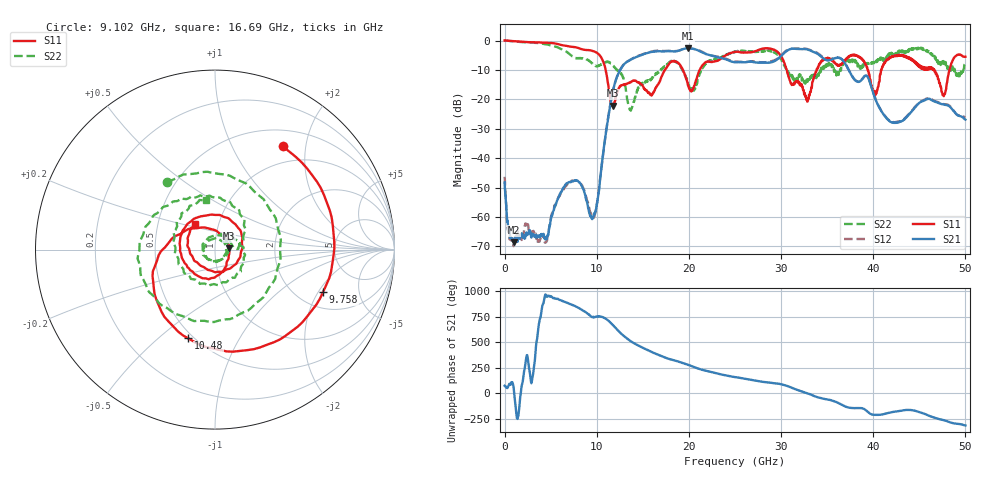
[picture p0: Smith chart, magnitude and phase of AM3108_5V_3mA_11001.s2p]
# Hz S DB R 50.0
!freq dBS11 angS11 dBS21 angS21 dBS12 angS12 dBS22 angS22
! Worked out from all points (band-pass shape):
!   1601 points, 10 MHz to 50 GHz, reference 50 ohm
!   highest |S21| = -2.67 dB at 19.91 GHz (marker M1); lowest = -68.6 dB at 978.6 MHz (marker M2)
!   |S21| within 3 dB of the highest: 14.24 GHz to 23.08 GHz (8.833 GHz wide, 47.3 % of centre); 29.86 GHz to 34.42 GHz (4.56 GHz wide, 14.2 % of centre)
!   lowest |S11| = -22.2 dB at 11.76 GHz (marker M3), VSWR 1.17, Z = 58.4 + j0.811 ohm
!   |S11| at or under -10 dB: 10.97 GHz to 17.4 GHz (6.428 GHz wide, 45.3 % of centre); 19.35 GHz to 21.17 GHz (1.819 GHz wide, 8.98 % of centre); 30.62 GHz to 33.85 GHz (3.227 GHz wide, 10 % of centre)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
!   |S22| runs from -23.9 to 0.0 dB; largest |S21 - S12| = 0.023
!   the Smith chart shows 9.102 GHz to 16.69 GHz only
!   S11 on the Smith chart (normalised r, x): 9.102 GHz: 0.73, +1.60; 9.758 GHz: 2.72, -2.21; 10.48 GHz: 0.47, -0.63; 16.69 GHz: 0.77, +0.23
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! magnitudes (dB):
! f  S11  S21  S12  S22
! 10 MHz  0.0  -48.2  -46.3  0.0
! 478.7 MHz  -0.1  -64.0  -65.4  -0.1
! 978.6 MHz  -0.2  -68.6  -69.9  -0.3
! 4.54 GHz  -0.8  -67.1  -68.4  -1.3
! 6.509 GHz  -1.7  -49.5  -49.8  -3.4
! 8.352 GHz  -2.9  -49.3  -49.0  -6.0
! 9.102 GHz  -3.3  -57.3  -55.8  -6.7
! 9.758 GHz  -3.8  -58.6  -59.7  -8.4
! 10.48 GHz  -5.7  -44.2  -44.2  -8.1
! 11.76 GHz  -22.2  -17.3  -17.2  -8.5
! 13.66 GHz  -14.3  -6.6  -6.5  -23.6
! 16.69 GHz  -14.7  -3.6  -3.4  -11.0
! 18.38 GHz  -7.0  -3.7  -3.6  -7.1
! 19.91 GHz  -15.3  -2.7  -2.6  -14.4
! 25 GHz  -3.9  -7.4  -7.2  -3.9
! 29.25 GHz  -3.1  -7.1  -6.8  -3.9
! 33.35 GHz  -15.7  -3.6  -3.4  -12.7
! 37.91 GHz  -4.9  -13.1  -13.0  -6.5
! 40.22 GHz  -18.7  -19.7  -19.6  -7.6
! 41.69 GHz  -6.1  -27.2  -27.0  -5.2
! 47.66 GHz  -18.9  -21.8  -21.6  -7.7
! 50 GHz  -5.5  -26.9  -26.1  -6.9
